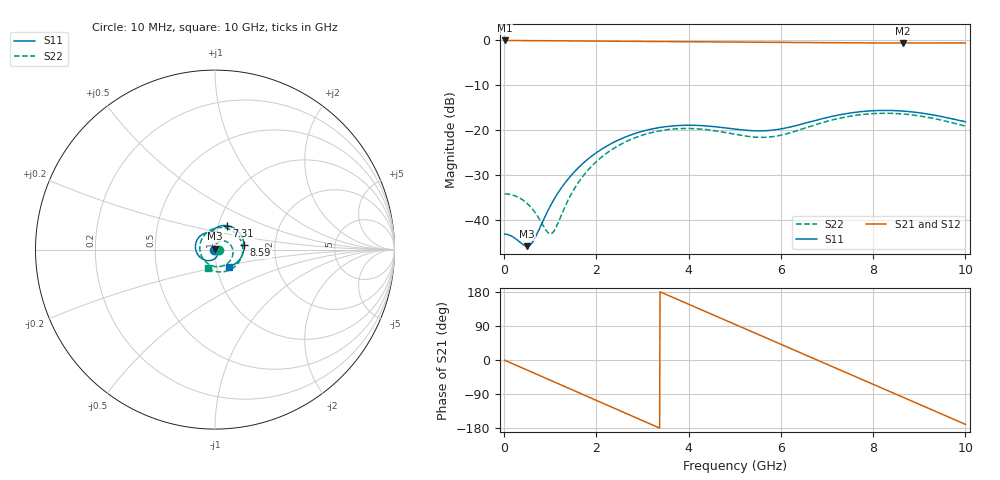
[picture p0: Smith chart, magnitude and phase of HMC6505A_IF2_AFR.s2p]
! Analog Devices, Inc.
! 1 Analog Way
! Wilmington, MA 01887
! http://www.analog.com
! Date:  2021-09-17 NN
! Board Name:  EV1HMC6505ALC5 (125487-1) with HMC6505ALC5 installed
! File Description:  Automatic Fixture Removal S-Parameters for IF2 Port connector and board loss de-embedding
! File Generation:  Calibrated Network Analyzer
! Chip Part Number:  HMC6505A
! Chip Description:  GaAs, MMIC, IQ Upconverter
! Chip Frequency:  5.5 to 8.6 GHz
! Chip Package:  LCC, 4.9 x 4.9 x 1 mm
! IF2 Port:  HMC6505ALC5 removed and end of trace left open
! Note:
!  Analog Devices supplies this data as a sample of measured data at the evaluation board
!  ports for this product.  Your particular data for this product may vary.
!  Analog Devices reserves the right to change this data at anytime.
!  All lines below in this file are as is from the Network Analyzer.
!Agilent Technologies,N5245A,MY52451809,A.10.47.06
!Automatic Fixture Removal (AFR)
!Date: Friday, September 17, 2021 3:13:36 AM
!S2P File: Measurements: S11,S21,S12,S22:
# MHz S  RI  R 50
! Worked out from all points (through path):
!   1000 points, 10 MHz to 10 GHz, reference 50 ohm
!   highest |S21| = 0.00 dB at 10 MHz (marker M1); lowest = -0.6 dB at 8.65 GHz (marker M2)
!   group delay of S21, straight-line fit = 147 ps
!   lowest |S11| = -45.8 dB at 500 MHz (marker M3), VSWR 1.01, Z = 50 + j0.509 ohm
!   |S11| at or under -10 dB: start of sweep to end of sweep
!   |S22| runs from -43.1 to -16.2 dB; largest |S21 - S12| = 1.4e-15
!   S11 on the Smith chart (normalised r, x): 10 MHz: 0.99, +0.00; 7.31 GHz: 1.10, +0.30; 8.59 GHz: 1.39, +0.07; 10 GHz: 1.15, -0.22
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10  -0.00697 0.000166  0.9997 -0.00932  0.9997 -0.00932  0.0195 -9.19e-05
500  0.000395 0.00509  0.8901 -0.4478  0.8901 -0.4478  0.015 -0.0028
650  0.00449 0.00405  0.8182 -0.5669  0.8182 -0.5669  0.0123 -0.00213
1030  0.014 -0.00605  0.5693 -0.8135  0.5693 -0.8135  0.00558 0.00434
1680  0.00849 -0.0405  0.00464 -0.9882  0.00464 -0.9882  0.00659 0.0287
2130  -0.0192 -0.0592  -0.3963 -0.9012  -0.3963 -0.9012  0.0244 0.0448
2610  -0.061 -0.0567  -0.7427 -0.6392  -0.7427 -0.6392  0.056 0.0472
3340  -0.1064 -0.00436  -0.972 -0.0341  -0.972 -0.0341  0.0975 0.00564
4080  -0.0946 0.0627  -0.7708 0.5828  -0.7708 0.5828  0.0811 -0.0655
4560  -0.0665 0.087  -0.4455 0.8536  -0.4455 0.8536  0.0329 -0.0931
5010  -0.0417 0.094  -0.0633 0.9579  -0.0633 0.9579  -0.0235 -0.0869
5370  -0.0284 0.0946  0.2521 0.9237  0.2521 0.9237  -0.062 -0.0572
5750  -0.0198 0.0973  0.5528 0.7783  0.5528 0.7783  -0.0835 -0.008
6230  -0.00874 0.109  0.8299 0.4639  0.8299 0.4639  -0.0718 0.0615
6670  0.012 0.1248  0.9421 0.098  0.9421 0.098  -0.0246 0.109
7310  0.0676 0.1335  0.8331 -0.4396  0.8331 -0.4396  0.0734 0.116
7850  0.1225 0.1075  0.5218 -0.7802  0.5218 -0.7802  0.138 0.0615
8340  0.1561 0.0565  0.1305 -0.928  0.1305 -0.928  0.1537 -0.0137
8590  0.1622 0.025  -0.0843 -0.933  -0.0843 -0.933  0.1433 -0.0516
8650  0.1624 0.0174  -0.1356 -0.927  -0.1356 -0.927  0.1391 -0.06
9250  0.1403 -0.0514  -0.603 -0.7178  -0.603 -0.7178  0.0695 -0.1182
10000  0.0807 -0.0944  -0.9241 -0.1643  -0.9241 -0.1643  -0.0374 -0.1046
